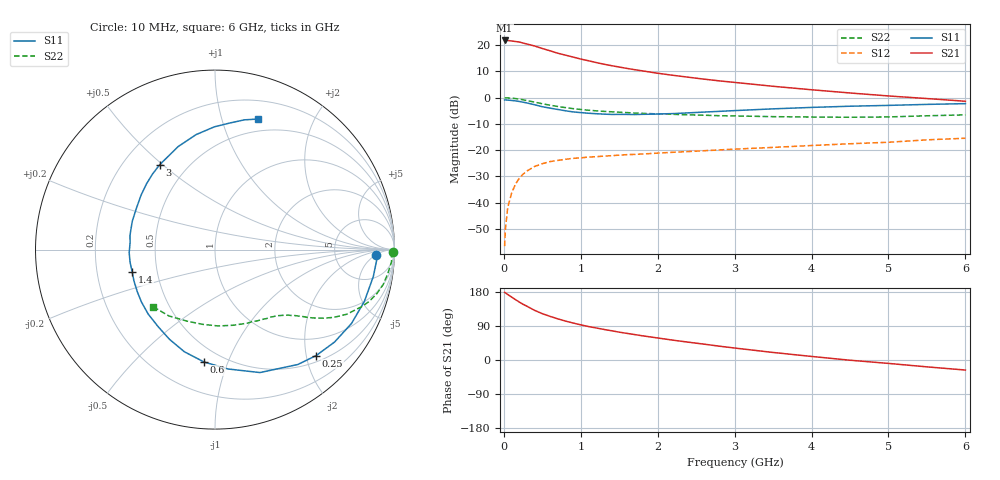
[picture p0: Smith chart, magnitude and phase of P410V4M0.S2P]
! SIEMENS Small Signal Semiconductors
! BFP182
! Si NPN RF Bipolar Junction Transistor in SOT143
! VCE = 10 V  IC = 4 mA
! Common Emitter S-Parameters:  March  1996
# GHz  S  MA  R  50
!  f  S11  S21  S12  S22
! GHz  MAG  ANG  MAG  ANG  MAG  ANG  MAG  ANG
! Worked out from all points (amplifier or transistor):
!   36 points, 10 MHz to 6 GHz, reference 50 ohm
!   highest |S21| = 21.7 dB at 10 MHz (marker M1)
!   |S21| within 3 dB of that: start of sweep to 494.6 MHz
!   unconditionally stable (mu >= 1): 1.839 GHz to 5.835 GHz
!   at 250 MHz: K = 0.18, MSG = 24.9 dB, |S12| = -29.1 dB
!   at 1.4 GHz: K = 0.84, MSG = 17.1 dB, |S12| = -22.1 dB
!   at 6 GHz: K = 0.98, MSG = 7.0 dB, |S12| = -15.5 dB
!   S11 on the Smith chart (normalised r, x): 10 MHz: 17, -5; 250 MHz: 0.62, -2.19; 600 MHz: 0.40, -0.83; 1.4 GHz: 0.36, -0.12; 3 GHz: 0.35, +0.49; 6 GHz: 0.37, +1.31
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0.01  0.8995 -1.8  12.15 178.4  0.0015 75.6  0.9895 -0.8
0.02  0.9025 -3.8  12.08 177.4  0.0031 80.3  0.9844 -1.6
0.05  0.8948 -9.6  12.15 172.9  0.0081 84.8  0.9859 -4.0
0.1  0.8809 -19.1  11.88 166.3  0.0151 78.8  0.9718 -8.0
0.2  0.842 -37.7  11.36 153.0  0.0291 68.9  0.9331 -15.4
0.25  0.8163 -46.3  10.84 147.0  0.0349 65.3  0.9061 -18.6
0.3  0.7892 -54.2  10.4 141.9  0.0402 60.7  0.8762 -21.3
0.4  0.7295 -69.9  9.523 131.0  0.049 54.2  0.8182 -26.1
0.5  0.669 -83.8  8.552 122.3  0.0553 48.4  0.7621 -29.7
0.6  0.6294 -95.5  7.734 115.2  0.0606 44.4  0.7151 -32.3
0.7  0.5942 -106.7  6.958 108.7  0.0639 41.4  0.6771 -34.3
0.8  0.5605 -116.9  6.391 102.8  0.0671 38.0  0.6439 -36.0
0.9  0.5334 -126.5  5.877 97.6  0.0699 36.5  0.6155 -37.3
1.1  0.5032 -144.5  5.004 88.3  0.074 33.4  0.5748 -39.7
1.4  0.4779 -164.9  4.033 77.2  0.0785 30.5  0.5363 -43.0
1.8  0.4801 170.6  3.216 63.9  0.0846 29.3  0.5009 -47.6
2.2  0.4951 152.0  2.644 52.3  0.0912 28.1  0.4801 -53.1
3  0.5647 123.0  1.94 31.6  0.1047 26.2  0.4473 -66.5
3.5  0.6095 109.7  1.635 19.9  0.1129 24.7  0.4334 -76.5
4.5  0.684 90.3  1.221 -0.6  0.1325 21.0  0.4221 -99.8
5.5  0.741 77.3  0.957 -18.1  0.1572 17.4  0.4502 -124.8
6  0.7657 71.8  0.85 -26.5  0.1686 13.6  0.4687 -137.2
